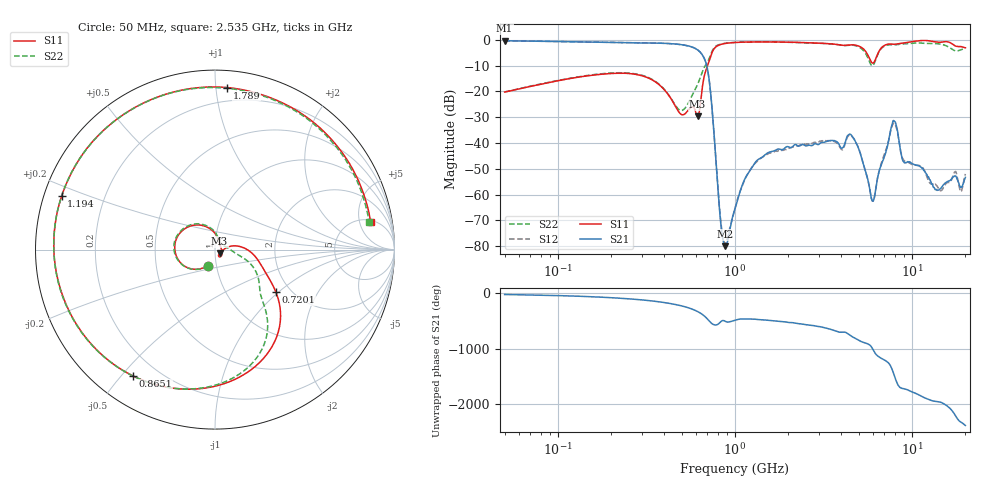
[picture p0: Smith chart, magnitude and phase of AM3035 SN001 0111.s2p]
# Hz S DB R 50
!freq MagS11 AngS11 MagS21 AngS21 MagS12 AngS12 MagS22 AngS22
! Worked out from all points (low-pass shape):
!   1601 points, 50 MHz to 20.05 GHz, reference 50 ohm
!   highest |S21| = -0.38 dB at 50 MHz (marker M1); lowest = -79.9 dB at 884.8 MHz (marker M2)
!   |S21| within 3 dB of the highest: start of sweep to 598 MHz
!   lowest |S11| = -29.7 dB at 615.2 MHz (marker M3), VSWR 1.07, Z = 52.6 - j2.17 ohm
!   |S11| at or under -10 dB: start of sweep to 701.1 MHz
!   |S22| runs from -27.4 to -0.8 dB; largest |S21 - S12| = 0.0046
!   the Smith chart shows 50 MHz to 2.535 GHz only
!   S11 on the Smith chart (normalised r, x): 50 MHz: 0.91, -0.17; 720.1 MHz: 1.68, -0.96; 865.1 MHz: 0.11, -0.54; 1.194 GHz: 0.05, +0.17; 1.789 GHz: 0.11, +1.07; 2.535 GHz: 5.39, +7.43
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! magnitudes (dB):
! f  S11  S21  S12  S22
! 50 MHz  -20.2  -0.4  -0.4  -20.2
! 135.9 MHz  -14.3  -0.8  -0.8  -14.1
! 369.6 MHz  -17.2  -1.3  -1.3  -17.0
! 496.9 MHz  -28.9  -1.9  -1.9  -27.4
! 615.2 MHz  -29.7  -3.9  -3.9  -17.3
! 678.2 MHz  -12.9  -7.9  -7.9  -10.1
! 720.1 MHz  -7.7  -17.1  -17.2  -6.8
! 824 MHz  -1.9  -68.2  -67.2  -1.8
! 865.1 MHz  -1.5  -79.0  -78.0  -1.4
! 884.8 MHz  -1.4  -79.9  -78.9  -1.3
! 1.005 GHz  -1.0  -65.1  -64.9  -1.0
! 1.194 GHz  -0.9  -51.5  -51.4  -0.9
! 1.789 GHz  -0.9  -42.4  -43.1  -0.9
! 2.535 GHz  -1.1  -41.1  -40.4  -1.2
! 2.722 GHz  -1.2  -41.0  -40.2  -1.3
! 4.565 GHz  -2.0  -37.2  -37.3  -2.1
! 6.024 GHz  -9.0  -62.5  -62.5  -9.9
! 7.402 GHz  -1.6  -38.7  -38.8  -1.9
! 7.978 GHz  -1.7  -31.6  -32.4  -2.0
! 9.028 GHz  -1.2  -47.5  -46.8  -1.6
! 14.42 GHz  -1.0  -57.8  -58.3  -1.6
! 20.05 GHz  -3.1  -53.3  -52.0  -3.6
